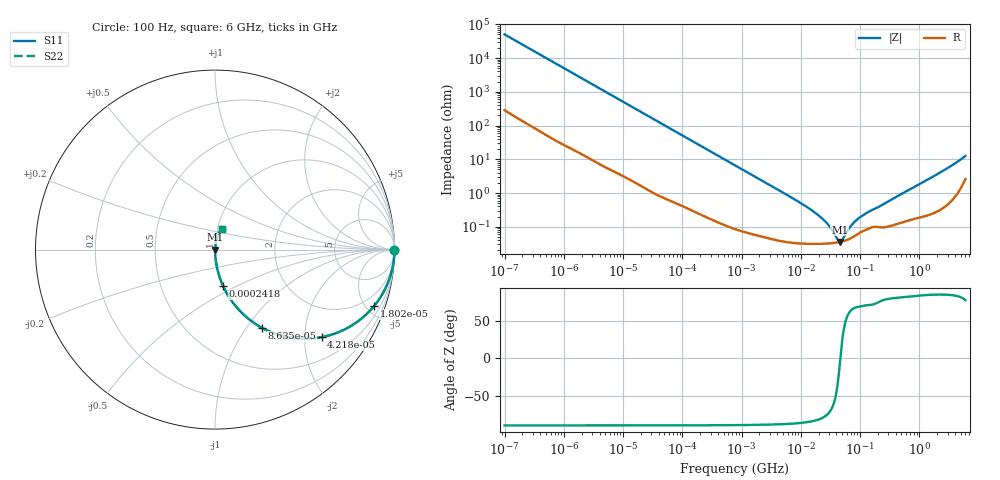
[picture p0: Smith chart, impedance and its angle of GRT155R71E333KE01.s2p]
!Murata Part Number: GRT155R71E333KE01
!These Parameters are Measured in Series Mode Connection
!Data Generated on Jun 19, 2026
!  o--ll--o
!Port1  Port2
!  o------o
!Operation Temp=25[degC], DC Bias Voltage=0[V]
!Freq. Start=100[Hz] Stop=6[GHz] 401[Steps]
# Hz S RI R 50
!Freq.(Hz) S11(Real) S11(Imag) S21(Real) S21(Imag) S12(Real) S12(Imag) S22(Real) S22(Imag)
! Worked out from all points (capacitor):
!   401 points, 100 Hz to 6 GHz, reference 50 ohm
!   read as one part in series: C = 31.8 nF near 109 Hz
!   lowest |Z| = 35.8 mohm at 45.56 MHz (marker M1)
!   series resonance near 46.48 MHz, so ESL is about 370 pH
!   S11 on the Smith chart (normalised r, x): 100 Hz: open; 18.02 kHz: 1.04, -5.65; 42.18 kHz: 1.02, -2.42; 86.35 kHz: 1.01, -1.19; 241.8 kHz: 1.00, -0.43; 6 GHz: 1.05, +0.25
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100  1 -0.002  1.55e-05 0.002  1.55e-05 0.002  1 -0.002
2008  0.9982 -0.0397  0.0018 0.0397  0.0018 0.0397  0.9982 -0.0397
6728  0.982 -0.1302  0.018 0.1302  0.018 0.1302  0.982 -0.1302
18016  0.8872 -0.3132  0.1128 0.3132  0.1128 0.3132  0.8872 -0.3132
26957  0.7801 -0.411  0.2199 0.411  0.2199 0.411  0.7801 -0.411
40335  0.615 -0.4833  0.385 0.4833  0.385 0.4833  0.615 -0.4833
42182  0.5938 -0.4878  0.4062 0.4878  0.4062 0.4878  0.5938 -0.4878
86348  0.2619 -0.4358  0.7381 0.4358  0.7381 0.4358  0.2619 -0.4358
141303  0.1187 -0.3192  0.8813 0.3192  0.8813 0.3192  0.1187 -0.3192
241822  0.0451 -0.2029  0.9549 0.2029  0.9549 0.2029  0.0451 -0.2029
774597  0.00529 -0.0664  0.9947 0.0664  0.9947 0.0664  0.00529 -0.0664
1.555665e7  0.00032 -0.003  0.9997 0.003  0.9997 0.003  0.00032 -0.003
2.662322e7  0.000319 -0.00133  0.9997 0.00133  0.9997 0.00133  0.000319 -0.00133
3.330331e7  0.000328 -0.000769  0.9997 0.000769  0.9997 0.000769  0.000328 -0.000769
4.165952e7  0.000345 -0.000248  0.9997 0.000248  0.9997 0.000248  0.000345 -0.000248
4.556224e7  0.000355 -4.47e-05  0.9996 4.47e-05  0.9996 4.47e-05  0.000355 -4.47e-05
4.983056e7  0.000368 0.000159  0.9996 -0.000159  0.9996 -0.000159  0.000368 0.000159
6.817316e7  0.000449 0.000887  0.9996 -0.000887  0.9996 -0.000887  0.000449 0.000887
9.326766e7  0.00063 0.00164  0.9994 -0.00164  0.9994 -0.00164  0.00063 0.00164
3.124326e8  0.00107 0.00584  0.9989 -0.00584  0.9989 -0.00584  0.00107 0.00584
1.95892e9  0.00399 0.0349  0.996 -0.0349  0.996 -0.0349  0.00399 0.0349
6e9  0.0393 0.1153  0.9607 -0.1153  0.9607 -0.1153  0.0393 0.1153
